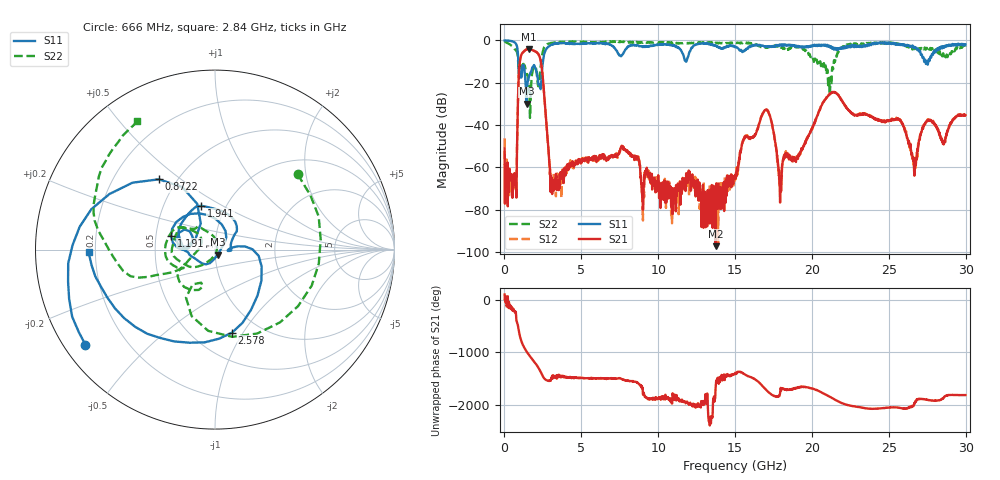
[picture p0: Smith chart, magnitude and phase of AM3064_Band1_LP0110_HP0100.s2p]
# Hz S DB R 50.0
!freq dBS11 angS11 dBS21 angS21 dBS12 angS12 dBS22 angS22
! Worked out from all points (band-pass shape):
!   1600 points, 10 MHz to 29.98 GHz, reference 50 ohm
!   highest |S21| = -4.09 dB at 1.584 GHz (marker M1); lowest = -97.1 dB at 13.73 GHz (marker M2)
!   |S21| within 3 dB of the highest: 1.085 GHz to 2.251 GHz (1.166 GHz wide, 69.9 % of centre)
!   lowest |S11| = -29.9 dB at 1.435 GHz (marker M3), VSWR 1.07, Z = 51.5 - j2.9 ohm
!   |S11| at or under -10 dB: 902.2 MHz to 2.506 GHz (1.603 GHz wide, 94.1 % of centre); 27.39391 GHz to 27.45908 GHz (65.17 MHz wide, 0.238 % of centre); 27.48961 GHz to 27.56275 GHz (73.14 MHz wide, 0.266 % of centre)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
!   |S22| runs from -36.6 to -0.4 dB; largest |S21 - S12| = 0.0068
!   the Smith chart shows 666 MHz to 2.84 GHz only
!   S11 on the Smith chart (normalised r, x): 666 MHz: 0.06, -0.33; 872.2 MHz: 0.40, +0.42; 1.191 GHz: 0.60, +0.10; 1.941 GHz: 0.77, +0.40; 2.578 GHz: 0.75, -0.90; 2.84 GHz: 0.17, -0.01
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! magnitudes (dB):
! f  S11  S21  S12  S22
! 10 MHz  0.0  -51.0  -46.3  -0.4
! 666 MHz  -1.0  -67.4  -67.7  -4.1
! 872.2 MHz  -6.0  -30.8  -30.7  -8.1
! 1.191 GHz  -11.8  -5.8  -5.7  -11.4
! 1.435 GHz  -29.9  -4.3  -4.3  -16.0
! 1.584 GHz  -17.3  -4.1  -4.1  -21.2
! 1.941 GHz  -11.8  -5.0  -5.0  -12.6
! 2.578 GHz  -6.5  -25.1  -25.2  -3.2
! 2.84 GHz  -3.0  -49.4  -49.5  -1.6
! 3.14 GHz  -1.8  -67.7  -68.0  -1.1
! 5.015 GHz  -1.4  -57.7  -56.8  -0.7
! 10 GHz  -2.0  -63.7  -70.7  -0.9
! 13.73 GHz  -2.5  -97.1  -70.6  -1.1
! 15 GHz  -3.0  -64.8  -65.9  -1.4
! 16.95 GHz  -2.7  -32.9  -32.8  -3.1
! 17.93 GHz  -2.1  -76.6  -71.4  -2.8
! 19.99 GHz  -2.9  -41.7  -42.0  -8.3
! 21.38 GHz  -3.3  -24.5  -24.6  -13.6
! 25 GHz  -1.0  -37.7  -37.7  -1.3
! 26.68 GHz  -3.1  -60.5  -59.6  -4.1
! 27.49 GHz  -9.9  -38.3  -37.9  -3.9
! 29.98 GHz  -1.9  -35.3  -35.2  -3.0
